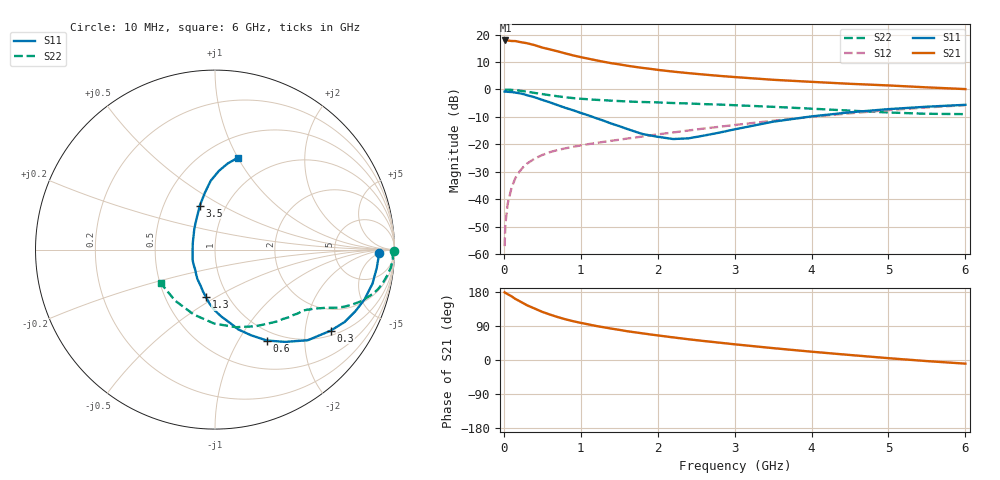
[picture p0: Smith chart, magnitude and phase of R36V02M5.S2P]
! SIEMENS Small Signal Semiconductors
! BFR181
! Si NPN RF Bipolar Junction Transistor in SOT23
! VCE = 6 V  IC = 2.5 mA
! Common Emitter S-Parameters:  May  1996
# GHz  S  MA  R  50
!  f  S11  S21  S12  S22
! GHz  MAG  ANG  MAG  ANG  MAG  ANG  MAG  ANG
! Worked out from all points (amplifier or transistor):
!   36 points, 10 MHz to 6 GHz, reference 50 ohm
!   highest |S21| = 17.9 dB at 20 MHz (marker M1)
!   |S21| within 3 dB of that: start of sweep to 560.6 MHz
!   unconditionally stable (mu >= 1): 1.513 GHz to 3.338 GHz
!   at 250 MHz: K = 0.26, MSG = 22.7 dB, |S12| = -28.3 dB
!   at 1.4 GHz: K = 0.97, MSG = 14.1 dB, |S12| = -18.7 dB
!   at 6 GHz: K = 0.86, MSG = 2.9 dB, |S12| = -5.7 dB
!   S11 on the Smith chart (normalised r, x): 10 MHz: 21, -5; 300 MHz: 1.15, -2.74; 600 MHz: 0.87, -1.33; 1.3 GHz: 0.79, -0.45; 3.5 GHz: 0.75, +0.40; 6 GHz: 0.71, +1.00
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0.01  0.9157 -1.3  7.724 178.6  0.0014 84.1  0.9959 -0.6
0.02  0.9129 -2.4  7.818 177.2  0.0035 91.7  0.9881 -1.2
0.05  0.9071 -6.4  7.812 173.7  0.0083 87.2  0.9925 -2.9
0.1  0.8978 -12.2  7.643 168.1  0.0162 83.4  0.9849 -5.8
0.15  0.8785 -18.3  7.622 161.1  0.0244 79.0  0.9695 -8.7
0.3  0.7871 -35.0  6.971 144.6  0.0445 70.5  0.9129 -15.7
0.4  0.7229 -44.3  6.427 135.8  0.0551 65.9  0.8661 -19.3
0.5  0.6465 -52.7  5.8 127.0  0.0641 62.9  0.824 -21.8
0.6  0.5831 -60.3  5.369 119.9  0.0723 60.3  0.7862 -23.9
0.7  0.5178 -67.2  4.953 113.3  0.079 59.0  0.7516 -25.5
0.8  0.4635 -73.7  4.538 107.5  0.0848 57.2  0.722 -26.7
0.9  0.4187 -78.2  4.18 102.4  0.0904 56.9  0.6974 -27.7
1.1  0.3371 -90.5  3.634 93.9  0.1011 56.2  0.6625 -29.6
1.3  0.2693 -100.8  3.19 86.3  0.1114 56.1  0.6364 -31.2
1.6  0.1916 -120.7  2.716 76.0  0.1276 56.9  0.6069 -33.7
1.9  0.1457 -144.9  2.381 67.6  0.1456 57.6  0.5866 -36.8
2.2  0.1252 -174.6  2.117 59.7  0.1648 57.9  0.5667 -40.2
2.8  0.1637 134.7  1.77 45.8  0.2092 56.8  0.5319 -48.6
3.5  0.2591 109.1  1.502 31.3  0.2693 53.3  0.4834 -62.1
4.5  0.3838 93.6  1.269 13.2  0.3685 44.8  0.4121 -90.6
5.5  0.4859 81.5  1.093 -2.9  0.4711 32.6  0.361 -128.0
6  0.526 76.2  1.017 -9.6  0.5186 25.5  0.3557 -148.6
